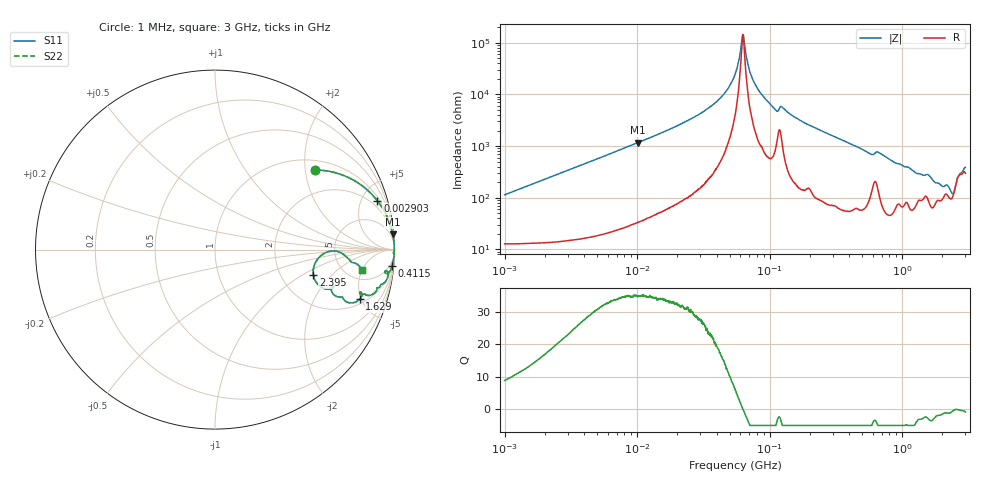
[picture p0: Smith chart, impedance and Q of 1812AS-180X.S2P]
!s-Parameter Generated by FASTRON Sdn. Bhd.
!FASTRON P/N : 1812AS-180X
!Keysight Technologies,E4991B,MY54100416,A.01.15
!Date created: Mon Oct 16 09:47:53 2023
!Version  : Rev00 Mon Oct 16 09:47:53 2023
!Data & Calibration Information:
!Freq	S11	S21	S12	S22
!PortZ  Port1:50+j0  Port2:50+j0
!When reading, reference impedance value at option line is always used.
! Remarks : This data is being provided solely for informational purposes.
# Hz S dB R 50
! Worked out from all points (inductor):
!   1601 points, 1 MHz to 3 GHz, reference 50 ohm
!   read as one part in series: L = 17.9 uH near 1.041 MHz
!   highest Q = 35.1 at 10.14 MHz (marker M1), where L = 18.2 uH
!   self-resonance near 62.7 MHz
!   S11 on the Smith chart (normalised r, x): 1 MHz: 1.25, +2.26; 2.903 MHz: 1.29, +6.55; 411.5 MHz: 2, -22; 1.629 GHz: 2.40, -4.87; 2.395 GHz: 3.03, -1.27; 3 GHz: 6.92, -5.01
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1000000  -2.95 38.5  -4.06 -45.0  -4.06 -45.0  -2.95 38.5
2903299  -0.49 16.7  -10.80 -70.7  -10.80 -70.7  -0.49 16.7
3804036  -0.30 13.0  -12.96 -74.9  -12.96 -74.9  -0.30 13.0
1.01436e7  -0.05 4.9  -21.36 -83.4  -21.36 -83.4  -0.05 4.9
1.447069e7  -0.03 3.4  -24.62 -84.9  -24.62 -84.9  -0.03 3.4
3.652005e7  -0.01 0.9  -35.63 -86.5  -35.63 -86.5  -0.01 0.9
4.6902e7  -0.01 0.5  -41.24 -85.0  -41.24 -85.0  -0.01 0.5
5.477226e7  -0.01 0.2  -47.71 -80.4  -47.71 -80.4  -0.01 0.2
5.787165e7  -0.01 0.1  -52.03 -74.4  -52.03 -74.4  -0.01 0.1
6.145316e7  -0.01 0.0  -60.31 -45.5  -60.31 -45.5  -0.01 0.0
6.301011e7  -0.01 -0.0  -63.19 4.8  -63.19 4.8  -0.01 -0.0
7.248696e7  -0.01 -0.2  -47.41 79.9  -47.41 79.9  -0.01 -0.2
8.766808e7  -0.01 -0.6  -39.84 83.8  -39.84 83.8  -0.01 -0.6
1.114693e8  -0.04 -1.1  -33.83 77.8  -33.83 77.8  -0.04 -1.1
1.244416e8  -0.03 -1.0  -35.11 78.0  -35.11 78.0  -0.03 -1.0
2.083556e8  -0.03 -2.3  -27.73 84.7  -27.73 84.7  -0.03 -2.3
4.114912e8  -0.08 -5.2  -20.82 81.9  -20.82 81.9  -0.08 -5.2
7.925923e8  -0.25 -9.9  -15.29 75.5  -15.29 75.5  -0.25 -9.9
1.629261e9  -1.38 -18.9  -9.45 55.1  -9.45 55.1  -1.38 -18.9
2.39512e9  -4.94 -14.5  -6.49 17.5  -6.49 17.5  -4.94 -14.5
2.568929e9  -3.50 -0.7  -9.59 1.4  -9.59 1.4  -3.50 -0.7
3e9  -1.64 -7.9  -13.42 32.3  -13.42 32.3  -1.64 -7.9
